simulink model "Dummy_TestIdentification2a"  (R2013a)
settings: Solver=ode45  StartTime=0  StopTime=5  FixedStep=1e-3  MaxStep=1e-3  RelTol=1e-6  AbsTol=1e-8
PreLoadFcn:
  | warning('off','sm:sli:setup:compile:LocalSolverNotSupported')
model workspace (MAT data in the model file):
  handle : class17 (value not decoded)
  handle : class17 (value not decoded)
undefined symbols (not defined in the file or in its folder): robotDen, robotNum, SimParam, var1

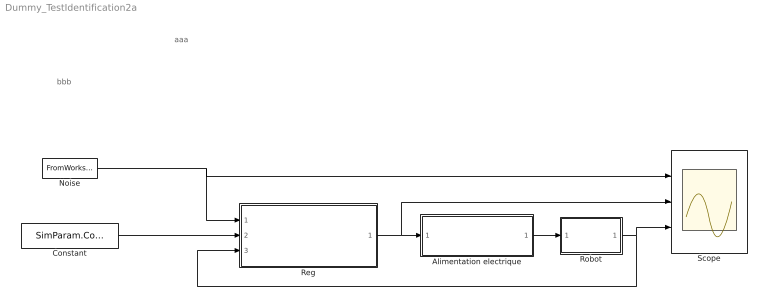
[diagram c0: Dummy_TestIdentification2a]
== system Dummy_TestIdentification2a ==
  note: aaa
  note: bbb
  Alimentation electrique : Subsystem
  Constant : Constant  Value=SimParam.CoderResol/1.5
  Noise : FromWorkspace  VariableName=Noise  SampleTime=SimParam.Te  Interpolate=off  OutputAfterFinalValue=Holding final value
  Reg : Subsystem
  Robot : Subsystem
  Scope : Scope  NumInputPorts=3
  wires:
  Noise/1 -> Reg/1(Noise), Scope/1
  Alimentation electrique/1(Torque_out) -> Robot/1(In1)
  Robot/1(Out1) -> Scope/3, Reg/3(Alpha)
  Reg/1(Torque) -> Scope/2, Alimentation electrique/1(Torque_in)
  Constant/1 -> Reg/2(Alpha_c)

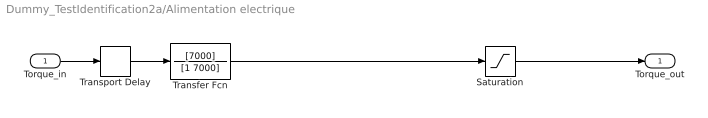
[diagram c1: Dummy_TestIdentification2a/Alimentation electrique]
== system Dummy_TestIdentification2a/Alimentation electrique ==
  Torque_in : Inport
  Saturation : Saturate  UpperLimit=20  LowerLimit=-20
  Transfer Fcn : TransferFcn  Numerator=[7000]  Denominator=[1 7000]
  Transport Delay : TransportDelay  DelayTime=150e-6
  Torque_out : Outport
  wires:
  Transfer Fcn/1 -> Saturation/1
  Torque_in/1 -> Transport Delay/1
  Saturation/1 -> Torque_out/1
  Transport Delay/1 -> Transfer Fcn/1

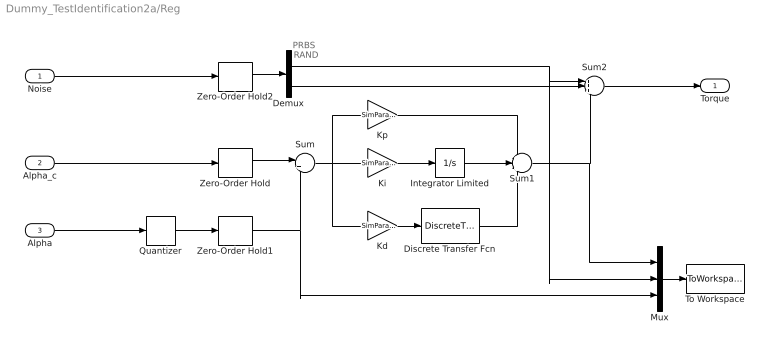
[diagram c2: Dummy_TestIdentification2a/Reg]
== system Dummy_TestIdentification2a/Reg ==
  note: RAND
  note: PRBS
  Noise : Inport
  Alpha_c : Inport  Port=2
  Alpha : Inport  Port=3
  Demux : Demux  Outputs=2
  Discrete Transfer Fcn : DiscreteTransferFcn  Numerator=[1 0 -1]  Denominator=[2 0 0]
  Integrator Limited : Integrator  LimitOutput=on  UpperSaturationLimit=1  LowerSaturationLimit=-1
  Kd : Gain  Gain=SimParam.Control.Kd/SimParam.Te
  Ki : Gain  Gain=SimParam.Control.Ki*SimParam.Te
  Kp : Gain  Gain=SimParam.Control.Kp
  Mux : Mux  Inputs=3
  Quantizer : Quantizer  QuantizationInterval=SimParam.CoderResol
  Sum : Sum  Inputs=|+-
  Sum1 : Sum  Inputs=+++
  Sum2 : Sum  Inputs=+++
  To Workspace : ToWorkspace  VariableName=simout  SaveFormat=Structure With Time  SampleTime=SimParam.Te
  Zero-Order Hold : ZeroOrderHold  SampleTime=SimParam.Te
  Zero-Order Hold1 : ZeroOrderHold  SampleTime=SimParam.Te
  Zero-Order Hold2 : ZeroOrderHold  SampleTime=SimParam.Te
  Torque : Outport
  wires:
  Alpha_c/1 -> Zero-Order Hold/1
  Kd/1 -> Discrete Transfer Fcn/1
  Mux/1 -> To Workspace/1
  Zero-Order Hold/1 -> Sum/1
  Sum/1 -> Ki/1, Kp/1, Kd/1
  Zero-Order Hold1/1 -> Sum/2, Mux/3
  Alpha/1 -> Quantizer/1
  Quantizer/1 -> Zero-Order Hold1/1
  Noise/1 -> Zero-Order Hold2/1
  Ki/1 -> Integrator Limited/1
  Discrete Transfer Fcn/1 -> Sum1/3
  Integrator Limited/1 -> Sum1/2
  Kp/1 -> Sum1/1
  Sum1/1 -> Mux/1, Sum2/3
  Zero-Order Hold2/1 -> Demux/1
  Demux/1 -> Mux/2, Sum2/1
  Demux/2 -> Sum2/2
  Sum2/1 -> Torque/1

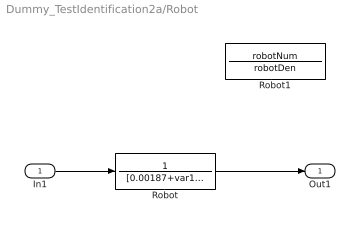
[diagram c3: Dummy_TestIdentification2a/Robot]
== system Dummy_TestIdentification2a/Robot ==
  In1 : Inport
  Robot : TransferFcn  Numerator=1  Denominator=[0.00187+var1 0 0]
  Robot1 : TransferFcn  Numerator=robotNum  Denominator=robotDen
  Out1 : Outport
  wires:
  In1/1 -> Robot/1
  Robot/1 -> Out1/1
